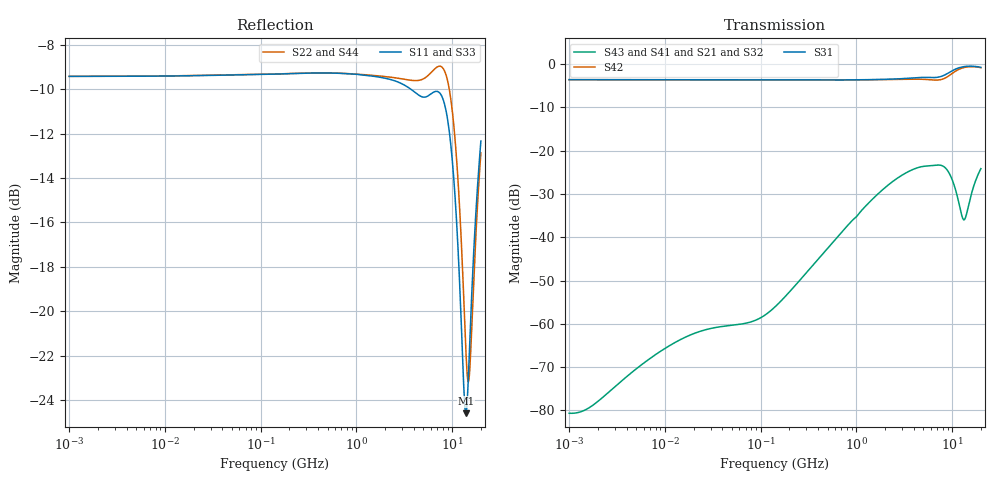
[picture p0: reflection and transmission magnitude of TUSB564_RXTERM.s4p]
! Created Tue Nov 01 10:37:03 2016
# hz S db R 50
! 4 Port Network Data from SP1.SP block
! freq  dbS11  angS11  dbS12  angS12  dbS13  angS13  dbS14  angS14
!  dbS21  angS21  dbS22  angS22  dbS23  angS23  dbS24  angS24
!  dbS31  angS31  dbS32  angS32  dbS33  angS33  dbS34  angS34
!  dbS41  angS41  dbS42  angS42  dbS43  angS43  dbS44  angS44
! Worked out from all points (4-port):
!   861 points, 1 MHz to 20 GHz, reference 50 ohm
!   strongest paths, dB at 1 MHz, 11.89 MHz, 141.4 MHz, 1.682 GHz, 20 GHz:
!     S31: -3.6, -3.6, -3.6, -3.5, -0.7
!     S42: -3.6, -3.6, -3.6, -3.6, -0.8
!     S43: -80.6, -64.7, -56.1, -30.0, -24.1
!     S41: -80.6, -64.7, -56.1, -30.0, -24.1
!     S21: -80.6, -64.7, -56.1, -30.0, -24.1
!     S32: -80.7, -64.8, -56.2, -30.0, -24.2
!   lowest |S11| = -24.6 dB at 14 GHz (marker M1), VSWR 1.13, Z = 44.5 - j1.12 ohm
!   |S11| at or under -10 dB: 3.73 GHz to end of sweep
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1000000  -9.41 -180.0  -80.69 17.0  -3.59 -0.0  -80.69 17.0
         -80.65 17.5  -9.41 -180.0  -80.65 17.5  -3.59 -0.0
         -3.59 -0.0  -80.69 17.0  -9.41 -180.0  -80.69 17.0
         -80.65 17.5  -3.59 -0.0  -80.65 17.5  -9.41 -180.0
1.549834e7  -9.39 -179.8  -63.44 49.4  -3.60 -0.1  -63.44 49.4
            -63.33 49.6  -9.38 -179.8  -63.33 49.6  -3.60 -0.1
            -3.60 -0.1  -63.44 49.4  -9.39 -179.8  -63.44 49.4
            -63.33 49.6  -3.60 -0.1  -63.33 49.6  -9.38 -179.8
1.123288e8  -9.32 -179.9  -58.04 67.5  -3.63 -0.0  -58.04 67.5
            -57.89 67.0  -9.32 -179.8  -57.89 67.0  -3.64 -0.1
            -3.63 -0.0  -58.04 67.5  -9.32 -179.9  -58.04 67.5
            -57.89 67.0  -3.64 -0.1  -57.89 67.0  -9.32 -179.8
3.596264e9  -9.95 170.4  -24.70 41.5  -3.24 4.4  -24.70 41.5
            -24.69 41.2  -9.58 175.5  -24.69 41.2  -3.48 2.2
            -3.24 4.4  -24.70 41.5  -9.95 170.4  -24.70 41.5
            -24.69 41.2  -3.48 2.2  -24.69 41.2  -9.58 175.5
8.82968e9  -11.17 150.2  -24.46 -16.8  -2.24 10.3  -24.46 -16.8
           -24.37 -16.7  -9.48 155.4  -24.37 -16.7  -2.99 11.4
           -2.24 10.3  -24.46 -16.8  -11.17 150.2  -24.46 -16.8
           -24.37 -16.7  -2.99 11.4  -24.37 -16.7  -9.48 155.4
1.399564e10  -24.60 -167.7  -35.02 31.8  -0.51 -0.8  -35.02 31.8
             -35.03 32.0  -21.92 162.0  -35.03 32.0  -0.69 1.5
             -0.51 -0.8  -35.02 31.8  -24.60 -167.7  -35.02 31.8
             -35.03 32.0  -0.69 1.5  -35.03 32.0  -21.92 162.0
2e10  -12.33 -116.5  -24.15 46.8  -0.74 -13.6  -24.15 46.8
      -24.15 46.7  -12.86 -119.5  -24.15 46.7  -0.82 -12.6
      -0.74 -13.6  -24.15 46.8  -12.33 -116.5  -24.15 46.8
      -24.15 46.7  -0.82 -12.6  -24.15 46.7  -12.86 -119.5
